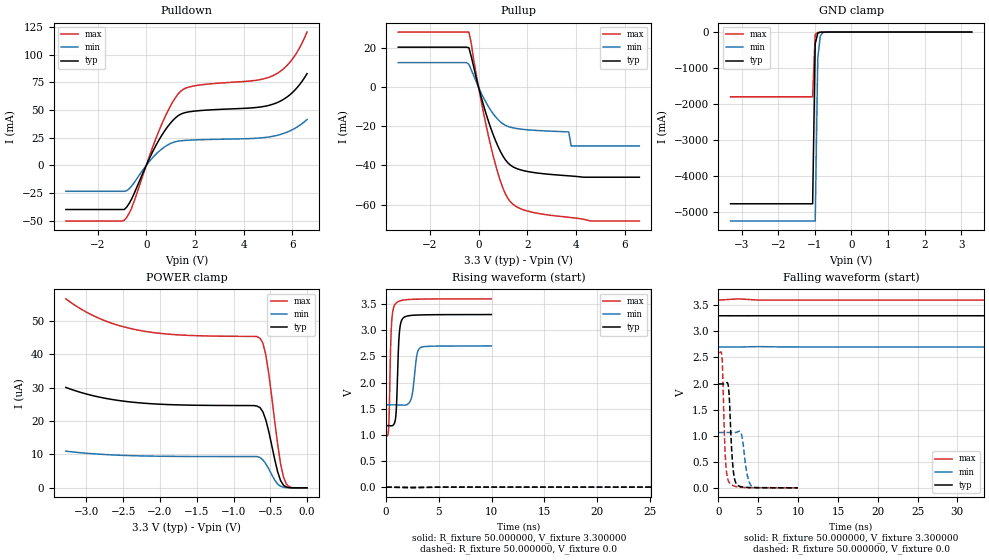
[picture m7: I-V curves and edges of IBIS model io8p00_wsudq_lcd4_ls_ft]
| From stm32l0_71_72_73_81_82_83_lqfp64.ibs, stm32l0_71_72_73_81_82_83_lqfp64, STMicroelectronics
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|   Model io8p00_wsudq_lcd4_ls_ft
[Model]  io8p00_wsudq_lcd4_ls_ft
Model_type I/O
Polarity   Non-Inverting
Enable   Active-Low
Vinl =   0.990000V
Vinh =   2.310000V
Vmeas =  1.650000V
Cref =   50.000000pF
Rref =   100.000000M
Vref =   0.0V
C_comp   3.263700pF   3.224700pF   3.309000pF
[Temperature Range]   25.000000   0.125000k   -40.000000
[Pullup Reference]   3.300000V   2.700000V   3.600000V
[Pulldown Reference]   0.0V   0.0V   0.0V
[POWER Clamp Reference]   3.300000V   2.700000V   3.600000V
[GND Clamp Reference]   0.0V   0.0V   0.0V
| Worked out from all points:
|   slope of the pulldown table from 0 to 0.495 V, typ, clamps not added: 22.6 ohm
|   slope of the pullup table from 0 to 0.495 V, typ, clamps not added: 23.9 ohm
|   GND clamp passes 1 mA (typ) near -0.64 V on its own axis
|   rising waveform, R_fixture 50.000000, V_fixture 3.300000: 20-80 % time 237ps typ, 378ps min, 201ps max; typ from 1.18 V to 3.3 V
|   rising waveform, R_fixture 50.000000, V_fixture 0.0: 20-80 % time 203ns typ, 423ns min, 99.3ns max; typ from 0 V to 1.99 V
|   falling waveform, R_fixture 50.000000, V_fixture 3.300000: 20-80 % time 191ns typ, 380ns min, 105ns max; typ from 3.3 V to 1.18 V
|   falling waveform, R_fixture 50.000000, V_fixture 0.0: 20-80 % time 414ps typ, 577ps min, 337ps max; typ from 1.99 V to 0 V
[Pulldown]
|Voltage   I(typ)   I(min)   I(max)
-3.3V     -39.83mA   -23.37mA   -50.2mA
-900mV    -39.83mA   -23.37mA   -49.52mA
-600mV    -30.28mA   -18.59mA   -38.45mA
500mV     22.11mA    12.28mA    30.1mA
1V        38.33mA    19.81mA    53.88mA
1.4V      46.1mA     22.18mA    66.72mA
2V        49.07mA    23.01mA    71.93mA
4.4V      52.05mA    24.38mA    76.53mA
5.2V      55.25mA    26.31mA    81.02mA
5.6V      59.18mA    28.57mA    86.57mA
6V        65.79mA    32.24mA    95.97mA
6.6V      82.83mA    41.41mA    120.4mA
[Pullup]
|Voltage   I(typ)   I(min)   I(max)
-3.3V     20.52mA    12.64mA    28.28mA
-400mV    20.25mA    11.77mA    28.28mA
-300mV    15.65mA    8.927mA    22.44mA
100mV     -4.685mA   -2.744mA   -6.647mA
600mV     -24.29mA   -13.56mA   -35.12mA
1V        -35.2mA    -18.69mA   -51.63mA
1.4V      -40.6mA    -20.72mA   -59.71mA
2.1V      -43.28mA   -21.83mA   -63.62mA
3.7V      -45.29mA   -22.8mA    -66.5mA
3.8V      -45.39mA   -30mA      -66.64mA
4.6V      -46mA      -30mA      -68.41mA
6.6V      -46mA      -30mA      -68.41mA
[GND_clamp]
|Voltage   I(typ)   I(min)   I(max)
-3.3V     -4.767A    -5.245A    -1.798A
-1.06V    -4.767A    -5.245A    -1.798A
-990mV    -327.3mA   -5.245A    -68.38mA
-920mV    -29.22mA   -722.7mA   -11.24mA
-850mV    -6.771mA   -104.4mA   -6.721mA
-780mV    -3.56mA    -17.38mA   -4.326mA
-500mV    -59.41uA   -172uA     -34.91uA
3.28V     0A         0A         0A
[POWER_clamp]
|Voltage   I(typ)   I(min)   I(max)
-3.28V    30.09uA    10.99uA    56.63uA
-2.84V    27.27uA    10.11uA    50.92uA
-2.32V    25.55uA    9.609uA    47.36uA
-640mV    24.06uA    9.1uA      44.84uA
-600mV    22.76uA    8.366uA    43.37uA
-560mV    20.32uA    7.212uA    39.74uA
-520mV    16.86uA    5.676uA    34.15uA
-400mV    4.842uA    1.146uA    13.11uA
-360mV    2.185uA    478.4nA    7.29uA
-320mV    773nA      181.6nA    3.214uA
-240mV    60.58nA    0A         296.5nA
0V        0A         0A         0A
[Ramp]
| variable   typ   min   max
dV/dt_r  1.19496/0.20321u   0.61278/0.42534u   1.55568/99.15978n
dV/dt_f  1.27296/0.19090u   0.63684/0.37991u   1.57856/0.10488u
R_load = 50.000000
[Rising Waveform]
R_fixture= 50.000000
V_fixture= 3.300000
V_fixture_min= 2.700000
V_fixture_max= 3.600000
|time   V(typ)   V(min)   V(max)
0s        1.177V     1.573V     967.4mV
240.2ps   1.176V     1.573V     1.138V
520.5ps   1.173V     1.574V     3.149V
860.9ps   1.277V     1.574V     3.502V
981ps     1.568V     1.574V     3.527V
1.241ns   2.921V     1.572V     3.556V
1.602ns   3.232V     1.568V     3.576V
2.362ns   3.283V     1.685V     3.59V
3.203ns   3.292V     2.661V     3.595V
9.97ns    3.3V       2.7V       3.6V
[Rising Waveform]
R_fixture= 50.000000
V_fixture= 0.0
V_fixture_min= 0.0
V_fixture_max= 0.0
|time   V(typ)   V(min)   V(max)
0s        2.524nV    17.58nV    5.69nV
50.05ns   679.3uV    -21.57uV   86.58mV
100.1ns   75.14mV    10.24uV    912.8mV
162.7ns   437.4mV    5.93mV     1.907V
202.7ns   729.3mV    14.45mV    2.277V
247.7ns   1.042V     47.15mV    2.469V
357.9ns   1.585V     189.6mV    2.573V
500.5ns   1.878V     438.1mV    2.59V
793.3ns   1.983V     848mV      2.592V
1.246us   1.992V     1.062V     2.592V
[Falling Waveform]
R_fixture= 50.000000
V_fixture= 3.300000
V_fixture_min= 2.700000
V_fixture_max= 3.600000
|time   V(typ)   V(min)   V(max)
0s        3.3V       2.7V       3.6V
82.58ns   3.3V       2.7V       3.491V
150.2ns   3.19V      2.7V       2.485V
212.7ns   2.837V     2.697V     1.574V
250.2ns   2.577V     2.686V     1.215V
285.3ns   2.324V     2.665V     1.08V
405.4ns   1.565V     2.53V      992.2mV
515.5ns   1.311V     2.339V     975.7mV
830.8ns   1.195V     1.784V     967.9mV
1.246us   1.177V     1.573V     967.4mV
[Falling Waveform]
R_fixture= 50.000000
V_fixture= 0.0
V_fixture_min= 0.0
V_fixture_max= 0.0
|time   V(typ)   V(min)   V(max)
0s        1.992V     1.062V     2.592V
440.4ps   1.992V     1.062V     2.508V
880.9ps   1.997V     1.062V     540.7mV
1.321ns   1.816V     1.062V     108.1mV
1.782ns   455mV      1.061V     47.51mV
2.282ns   69.45mV    1.068V     21.11mV
2.863ns   21.01mV    1.037V     8.711mV
3.624ns   7.551mV    238.3mV    4.508mV
4.164ns   4.362mV    34.44mV    3.282mV
9.97ns    2.524nV    17.58nV    5.69nV
